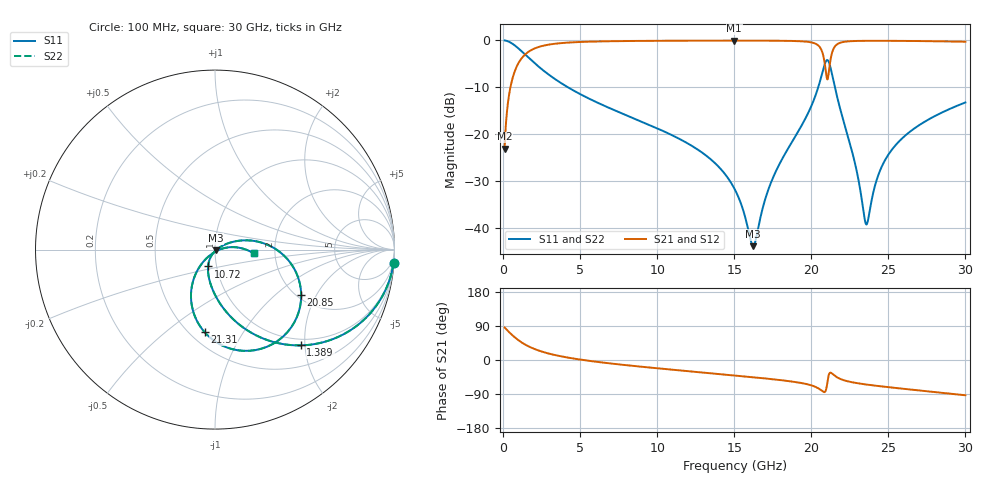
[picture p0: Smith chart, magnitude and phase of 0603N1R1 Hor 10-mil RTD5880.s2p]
# GHz S MA R 50
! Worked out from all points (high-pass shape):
!   3201 points, 100 MHz to 30 GHz, reference 50 ohm
!   highest |S21| = -0.05 dB at 15 GHz (marker M1); lowest = -23.1 dB at 100 MHz (marker M2)
!   |S21| within 3 dB of the highest: 1.417 GHz to 20.76 GHz (19.34 GHz wide, 174 % of centre); 21.32 GHz to end of sweep
!   lowest |S11| = -43.9 dB at 16.23 GHz (marker M3), VSWR 1.01, Z = 50.4 - j0.475 ohm
!   |S11| at or under -10 dB: 4.201 GHz to 20.45 GHz (16.25 GHz wide, 132 % of centre); 21.53 GHz to end of sweep
!   |S22| runs from -43.9 to 0.0 dB; largest |S21 - S12| = 0
!   S11 on the Smith chart (normalised r, x): 100 MHz: 1, -27; 1.389 GHz: 0.87, -1.92; 10.72 GHz: 0.91, -0.17; 20.85 GHz: 2.12, -1.51; 21.31 GHz: 0.59, -0.69; 30 GHz: 1.55, -0.07
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0.1  0.9975 -4.3  0.06972 85.7  0.06972 85.7  0.9975 -4.3
0.5671875  0.9295 -23.2  0.3683 66.7  0.3683 66.7  0.9295 -23.2
1.389438  0.7165 -48.1  0.6965 41.8  0.6965 41.8  0.7165 -48.1
2.791  0.4529 -70.9  0.8897 18.9  0.8897 18.9  0.4529 -70.9
5.089563  0.2624 -88.8  0.9623 0.6  0.9623 0.6  0.2624 -88.8
10.06978  0.1139 -110.1  0.9894 -22.1  0.9894 -22.1  0.1139 -110.1
10.72384  0.1017 -112.3  0.9905 -24.6  0.9905 -24.6  0.1017 -112.3
13.41484  0.05487 -119.5  0.9933 -34.7  0.9933 -34.7  0.05487 -119.5
15.00328  0.02634 -118.3  0.9938 -40.7  0.9938 -40.7  0.02634 -118.3
15.05  0.02546 -118.0  0.9938 -40.9  0.9938 -40.9  0.02546 -118.0
16.22731  0.006372 -47.7  0.9934 -45.5  0.9934 -45.5  0.006372 -47.7
17.47938  0.03316 26.0  0.9916 -50.7  0.9916 -50.7  0.03316 26.0
20.03956  0.2057 14.2  0.9485 -67.3  0.9485 -67.3  0.2057 14.2
20.55347  0.3599 -1.9  0.8461 -77.3  0.8461 -77.3  0.3599 -1.9
20.85247  0.5418 -27.6  0.5963 -84.8  0.5963 -84.8  0.5418 -27.6
21.09541  0.6069 -66.5  0.4081 -46.2  0.4081 -46.2  0.6069 -66.5
21.31031  0.4632 -97.2  0.6984 -34.6  0.6984 -34.6  0.4632 -97.2
22.00175  0.1558 -129.9  0.9557 -51.9  0.9557 -51.9  0.1558 -129.9
23.54347  0.01099 -70.6  0.9888 -64.5  0.9888 -64.5  0.01099 -70.6
24.30966  0.03503 5.7  0.9896 -68.5  0.9896 -68.5  0.03503 5.7
25.01978  0.06097 9.7  0.9888 -71.8  0.9888 -71.8  0.06097 9.7
30  0.2175 -5.6  0.9662 -93.1  0.9662 -93.1  0.2175 -5.6
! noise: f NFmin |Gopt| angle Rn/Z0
0.1  0.001691  0.9856  0.375  0.02679
3.417  0.004064  0.8115  10.33  0.00446
6.743  0.006804  0.7823  19.63  0.006229
10.06  0.009352  0.7675  28.84  0.007686
13.39  0.01199  0.7621  37.92  0.009168
16.7  0.01548  0.7716  46.75  0.01169
20.03  0.03599  0.877  55.45  0.04958
23.35  0.02363  0.7942  64.11  0.01713
26.67  0.02199  0.7564  72.16  0.01205
30  0.02426  0.7555  80.01  0.01193
